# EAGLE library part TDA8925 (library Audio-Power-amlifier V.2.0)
The TDA8925 is a switching power stage for a high efficiency class-D audio power amplifier system. With this power stage a compact 2 ´ 15 W self oscillating digital amplifier system can be built, operating with high efficiency and very low dissipation. No heatsink is required. The system operates over a wide supply voltage range from ±7.5 V up to ±30 V and consumes a very low quiescent current.
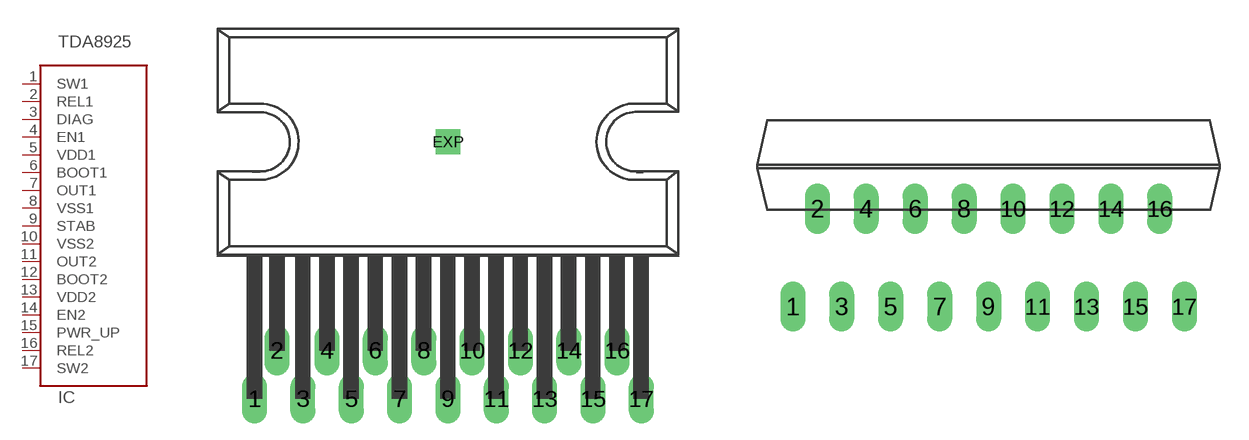
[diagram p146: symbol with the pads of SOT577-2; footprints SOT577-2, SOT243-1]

Designator prefix IC

## TDA8925  [SOT577-2]
1  SW1  in
2  REL1  out
3  DIAG  out
4  EN1  in
5  VDD1  pwr
6  BOOT1
7  OUT1  out
8  VSS1  pwr
9  STAB
10  VSS2  pwr
11  OUT2  out
12  BOOT2
13  VDD2  pwr
14  EN2  in
15  PWR_UP  in
16  REL2  out
17  SW2  in

## TDA8925SOT243  [SOT243-1]
Pads as for SOT577-2

## Footprint SOT577-2 (pad centres in mm)
drill 0.8 long: 1 -10.16,-13.5; 2 -8.98,-10.96; 3 -7.62,-13.5; 4 -6.35,-10.96; 5 -5.08,-13.5; 6 -3.81,-10.96; 7 -2.54,-13.5; 8 -1.27,-10.96; 9 0,-13.5; 10 1.27,-10.96; 11 2.54,-13.5; 12 3.81,-10.96; 13 5.08,-13.5; 14 6.35,-10.96; 15 7.62,-13.5; 16 8.89,-10.96; 17 10.16,-13.5
drill 0.8 square: EXP 0,0

## Footprint SOT243-1 (pad centres in mm)
DBS17P: plastic DIL-bent-SIL power package; 17 leads (lead length 7.7 mm)
drill 0.8 long: 1 -10.16,-5.08; 2 -8.89,0; 3 -7.62,-5.08; 4 -6.35,0; 5 -5.08,-5.08; 6 -3.81,0; 7 -2.54,-5.08; 8 -1.27,0; 9 0,-5.08; 10 1.27,0; 11 2.54,-5.08; 12 3.81,0; 13 5.08,-5.08; 14 6.35,0; 15 7.62,-5.08; 16 8.89,0; 17 10.17,-5.08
